FUNCTION_BLOCK "Div_Real"
VERSION : 0.1
   VAR_INPUT
      "I0.0" : Real;
      "I0.1" : Real;
   END_VAR

   VAR_OUTPUT
      "O0.0" : Real;
   END_VAR


BEGIN
NETWORK
TITLE =
      L #"I0.0";
      L #"I0.1";
      /R;
      T #"O0.0";
      NOP 0;
NETWORK
TITLE =
END_FUNCTION_BLOCK

